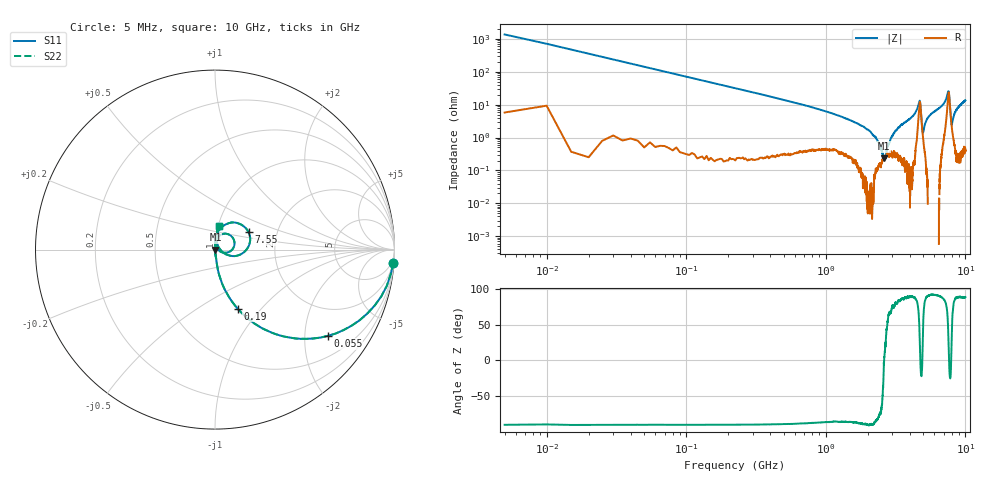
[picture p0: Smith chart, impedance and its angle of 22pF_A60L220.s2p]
! Amotech Co.,Ltd.
! http://www.amotech.co.kr/
! Part Number: A60L220
! These Parameters are Measured in Series Mode Connection
! Operation Temp=25[degC], DC Bias Voltage=0[V]
! Freq. Start=5[MHz] Stop=10[GHz], 2000[Steps]
! Date: Monday, July 14, 2020, 09:37:41
# GHZ S RI R 50.000000
!Freq.(Hz) S11(Real) S11(Imag) S21(Real) S21(Imag) S12(Real) S12(Imag) S22(Real) S22(Imag)
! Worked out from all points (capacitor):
!   2000 points, 5 MHz to 10 GHz, reference 50 ohm
!   read as one part in series: C = 22.2 pF near 55 MHz
!   lowest |Z| = 234 mohm at 2.615 GHz (marker M1)
!   series resonance near 2.616 GHz, so ESL is about 170 pH
!   S11 on the Smith chart (normalised r, x): 5 MHz: 1, -27; 55 MHz: 1.01, -2.60; 190 MHz: 1.00, -0.75; 7.55 GHz: 1.43, +0.29; 10 GHz: 1.01, +0.27
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0.005  0.9943 -0.0731  0.00569 0.0731  0.00569 0.0731  0.9943 -0.0731
0.055  0.6283 -0.4805  0.3717 0.4805  0.3717 0.4805  0.6283 -0.4805
0.1  0.3391 -0.4712  0.6609 0.4712  0.6609 0.4712  0.3391 -0.4712
0.19  0.1255 -0.3288  0.8745 0.3288  0.8745 0.3288  0.1255 -0.3288
0.645  0.0148 -0.1042  0.9852 0.1042  0.9852 0.1042  0.0148 -0.1042
1.675  0.00244 -0.027  0.9976 0.027  0.9976 0.027  0.00244 -0.027
2.28  0.00124 -0.00986  0.9988 0.00986  0.9988 0.00986  0.00124 -0.00986
2.615  0.00233 -2.11e-05  0.9977 2.11e-05  0.9977 2.11e-05  0.00233 -2.11e-05
2.95  0.00355 0.00948  0.9964 -0.00948  0.9964 -0.00948  0.00355 0.00948
3.34  0.00282 0.0205  0.9972 -0.0205  0.9972 -0.0205  0.00282 0.0205
4.24  0.00395 0.0467  0.9961 -0.0467  0.9961 -0.0467  0.00395 0.0467
4.69  0.0962 0.0694  0.9038 -0.0694  0.9038 -0.0694  0.0962 0.0694
4.765  0.0864 -0.00831  0.9136 0.00831  0.9136 0.00831  0.0864 -0.00831
4.92  0.0156 0.000715  0.9844 -0.000715  0.9844 -0.000715  0.0156 0.000715
5.005  0.00762 0.0134  0.9924 -0.0134  0.9924 -0.0134  0.00762 0.0134
5.49  0.00157 0.045  0.9984 -0.045  0.9984 -0.045  0.00157 0.045
6.67  0.00924 0.0855  0.9908 -0.0855  0.9908 -0.0855  0.00924 0.0855
7.55  0.1871 0.0969  0.8129 -0.0969  0.8129 -0.0969  0.1871 0.0969
7.67  0.1466 -0.0244  0.8534 0.0244  0.8534 0.0244  0.1466 -0.0244
7.96  0.0228 0.00919  0.9772 -0.00919  0.9772 -0.00919  0.0228 0.00919
8.335  0.00844 0.0506  0.9916 -0.0506  0.9916 -0.0506  0.00844 0.0506
10  0.0218 0.132  0.9782 -0.132  0.9782 -0.132  0.0218 0.132
